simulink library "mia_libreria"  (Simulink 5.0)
undefined symbols (not defined in the file or in its folder): contributo_inerzia, coriolis, gravload, ikine_rrprrr, ikine_rrprrr1, interp_cubica, interp_grado5, interp_punti_intermedi, matrice2vettore, spazio_di_lavoro, stanf, verifica_assestamento, vettore2matrice, xyzrpr2tr
libraries: mia_libreria x11, roblocks x2, simulink x1

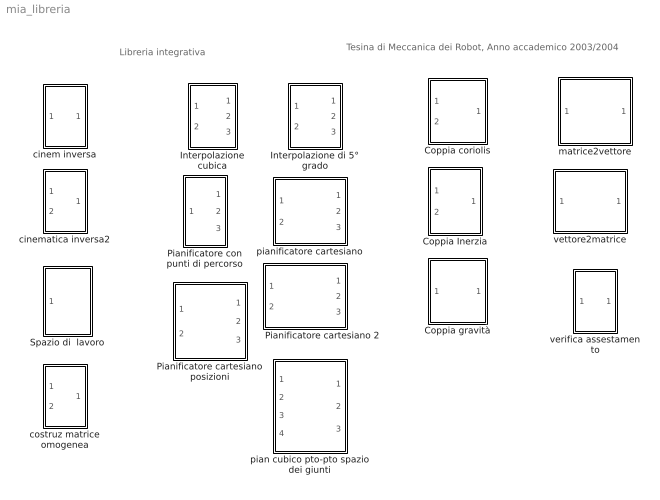
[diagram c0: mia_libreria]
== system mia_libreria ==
  note: Libreria integrativa
  note: Tesina di Meccanica dei Robot, Anno accademico 2003/2004
  Coppia Inerzia : Subsystem  mask{robot=0}
      mask prompts: robot "nome robot"
  Coppia coriolis : Subsystem  mask{robot=nome robot}
      mask prompts: robot "Variabile robot"
  Coppia gravità : Subsystem  mask{robot=0}
      mask prompts: robot "nome robot"
  Interpolazione cubica : Subsystem  mask{n=6, tf=1}
      mask prompts: n "dimensione uscita"; tf "tempo finale"
  Interpolazione di 5° grado : Subsystem  mask{n=0, tf=0}
      mask prompts: n "dimensione uscita"; tf "tempo finale"
  Pianificatore cartesiano 2 : Subsystem  mask{robot=0}
      mask prompts: robot "nome robot"
  Pianificatore cartesiano posizioni : Subsystem  mask{robot=stanf}
      mask prompts: robot "nome robot"
      mask help: funziona solo con manipolatori in cui il posizionamento dipende solo dalle variabili q1,q2,q3 e l'orientamento solo dalle variabili q4,q5,q6
  Pianificatore con punti di percorso : Subsystem  mask{robot=stanf, n_punti=2}
      mask prompts: robot "nome robot"; n_punti "numero punti traiettoria"
  Spazio di  lavoro : Subsystem  mask{robot=0}
      mask prompts: robot "nome robot"
  cinem inversa : Subsystem  mask{robot=stanf}
  cinematica inversa2 : Subsystem  mask{robot=stanf}
      mask prompts: robot "nome robot"
  costruz matrice omogenea : Subsystem
  matrice2vettore : Subsystem  mask{n_elementi=4}
      mask prompts: n_elementi "numero elementi della matrice"
  pian cubico pto-pto spazio dei giunti : Subsystem  mask{robot=0, tf=0}
      mask prompts: robot "nome robot"; tf "tempo finale"
  pianificatore cartesiano : Subsystem  mask{robot=0}
      mask prompts: robot "nome robot"
  verifica assestamento : Subsystem  mask{robot=stanf, vregime=1, scostpercentuale=0.1}
      mask prompts: robot "nome robot"; vregime "valore di regime desiderato"; scostpercentuale "scostamento dal valore di regime"
  vettore2matrice : Subsystem  mask{n_righe=2, n_colonne=2}
      mask prompts: n_righe "numero righe matrice uscita"; n_colonne "numero colonne matrice uscita"

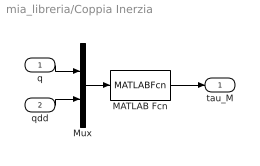
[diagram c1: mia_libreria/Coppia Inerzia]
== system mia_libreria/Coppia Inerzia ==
  q : Inport  PortDimensions=robot.n
  qdd : Inport  Port=2  PortDimensions=robot.n
  MATLAB Fcn : MATLABFcn  MATLABFcn=contributo_inerzia(robot,u(1:robot.n)',u(robot.n+1:2*robot.n)')  OutputDimensions=robot.n
  Mux : Mux  Inputs=2
  tau_M : Outport
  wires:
  Mux/1 -> MATLAB Fcn/1
  MATLAB Fcn/1 -> tau_M/1
  qdd/1 -> Mux/2
  q/1 -> Mux/1

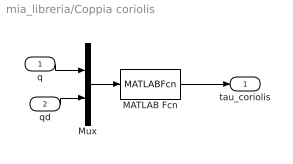
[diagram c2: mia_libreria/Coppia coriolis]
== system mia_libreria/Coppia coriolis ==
  q : Inport
  qd : Inport  Port=2
  MATLAB Fcn : MATLABFcn  MATLABFcn=coriolis(robot,u(1:robot.n)',u(robot.n+1:2*robot.n)')  OutputDimensions=robot.n
  Mux : Mux  Inputs=2
  tau_coriolis : Outport
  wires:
  Mux/1 -> MATLAB Fcn/1
  MATLAB Fcn/1 -> tau_coriolis/1
  qd/1 -> Mux/2
  q/1 -> Mux/1

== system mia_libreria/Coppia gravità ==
  q : Inport  PortDimensions=robot.n
  MATLAB Fcn : MATLABFcn  MATLABFcn=gravload(robot,u')  OutputDimensions=robot.n
  tau_grav : Outport
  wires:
  MATLAB Fcn/1 -> tau_grav/1
  q/1 -> MATLAB Fcn/1

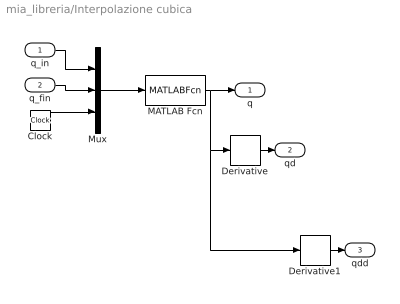
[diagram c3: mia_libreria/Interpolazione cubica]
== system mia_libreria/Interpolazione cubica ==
  q_in : Inport
  q_fin : Inport  Port=2
  Clock : Clock
  Derivative : Derivative
  Derivative1 : Derivative
  MATLAB Fcn : MATLABFcn  MATLABFcn=interp_cubica(u(1:n),u(n+1:2*n),tf,u(2*n+1))  OutputDimensions=n
  Mux : Mux  Inputs=3
  q : Outport
  qd : Outport  Port=2
  qdd : Outport  Port=3
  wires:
  MATLAB Fcn/1 -> q/1, Derivative/1, Derivative1/1
  q_in/1 -> Mux/1
  q_fin/1 -> Mux/2
  Clock/1 -> Mux/3
  Mux/1 -> MATLAB Fcn/1
  Derivative/1 -> qd/1
  Derivative1/1 -> qdd/1

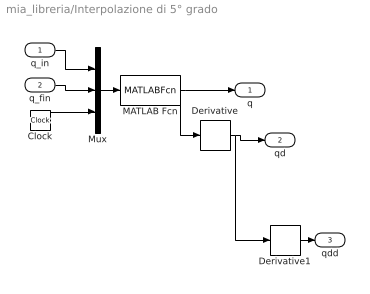
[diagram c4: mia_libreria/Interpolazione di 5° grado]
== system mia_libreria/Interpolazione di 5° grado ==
  q_in : Inport
  q_fin : Inport  Port=2
  Clock : Clock
  Derivative : Derivative
  Derivative1 : Derivative
  MATLAB Fcn : MATLABFcn  MATLABFcn=interp_grado5(u(1:n),u(n+1:2*n),tf,u(2*n+1))  OutputDimensions=n
  Mux : Mux  Inputs=3
  q : Outport
  qd : Outport  Port=2
  qdd : Outport  Port=3
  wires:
  Mux/1 -> MATLAB Fcn/1
  Clock/1 -> Mux/3
  q_fin/1 -> Mux/2
  q_in/1 -> Mux/1
  MATLAB Fcn/1 -> q/1, Derivative/1
  Derivative/1 -> qd/1, Derivative1/1
  Derivative1/1 -> qdd/1

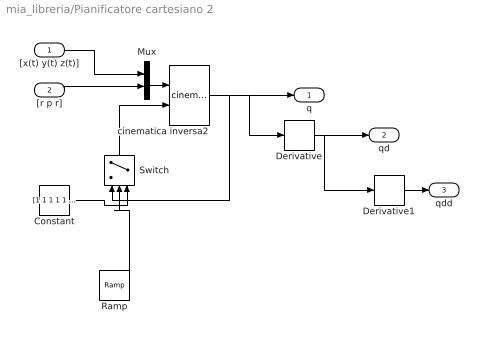
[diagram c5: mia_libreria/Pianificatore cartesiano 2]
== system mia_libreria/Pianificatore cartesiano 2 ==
  "[x(t) y(t) z(t)]" : Inport
  "[r p r]" : Inport  Port=2
  Constant : Constant  Value=[1 1 1 1 1 1]
  Derivative : Derivative
  Derivative1 : Derivative
  Mux : Mux  Inputs=2
  Ramp : simulink/Sources/Ramp  slope=1  start=0  X0=0
  Switch : Switch  Orientation=up  Threshold=1
  cinematica inversa2 : mia_libreria/cinematica inversa2  robot=stanf
  q : Outport
  qd : Outport  Port=2
  qdd : Outport  Port=3
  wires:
  Mux/1 -> cinematica inversa2/1
  "[r p r]"/1 -> Mux/2
  "[x(t) y(t) z(t)]"/1 -> Mux/1
  Derivative1/1 -> qdd/1
  Derivative/1 -> Derivative1/1, qd/1
  cinematica inversa2/1 -> Derivative/1, q/1, Switch/1
  Ramp/1 -> Switch/2
  Switch/1 -> cinematica inversa2/2
  Constant/1 -> Switch/3

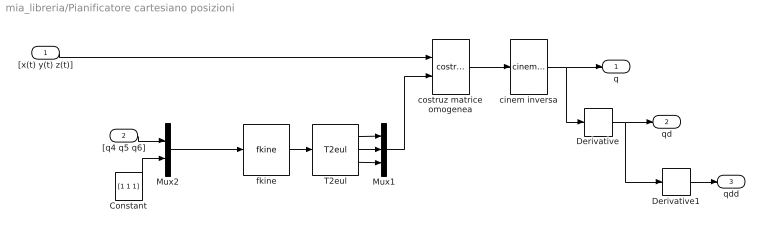
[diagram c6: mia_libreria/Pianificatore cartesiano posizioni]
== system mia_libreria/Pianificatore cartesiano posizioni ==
  "[x(t) y(t) z(t)]" : Inport
  "[q4 q5 q6]" : Inport  Port=2
  Constant : Constant  Value=[1 1 1]
  Derivative : Derivative
  Derivative1 : Derivative
  Mux1 : Mux  Inputs=3
  Mux2 : Mux  Inputs=2
  T2eul : roblocks/T2eul
  cinem inversa : mia_libreria/cinem inversa  robot=robot
  costruz matrice omogenea : mia_libreria/costruz matrice omogenea  SimViewingDevice=off  DataTypeOverride=UseLocalSettings  MinMaxOverflowLogging=UseLocalSettings
  fkine : roblocks/fkine  robot=robot
  q : Outport
  qd : Outport  Port=2
  qdd : Outport  Port=3
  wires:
  cinem inversa/1 -> q/1, Derivative/1
  Mux2/1 -> fkine/1
  Constant/1 -> Mux2/2
  "[q4 q5 q6]"/1 -> Mux2/1
  costruz matrice omogenea/1 -> cinem inversa/1
  Mux1/1 -> costruz matrice omogenea/2
  T2eul/3 -> Mux1/3
  T2eul/2 -> Mux1/2
  T2eul/1 -> Mux1/1
  fkine/1 -> T2eul/1
  "[x(t) y(t) z(t)]"/1 -> costruz matrice omogenea/1
  Derivative/1 -> qd/1, Derivative1/1
  Derivative1/1 -> qdd/1

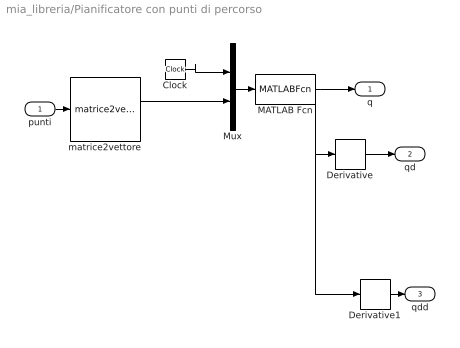
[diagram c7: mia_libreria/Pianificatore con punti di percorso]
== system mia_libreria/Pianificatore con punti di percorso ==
  punti : Inport
  Clock : Clock
  Derivative : Derivative
  Derivative1 : Derivative
  MATLAB Fcn : MATLABFcn  MATLABFcn=interp_punti_intermedi(vettore2matrice(u(2:n_punti*(2*robot.n+1)+1),n_punti,2*robot.n+1),u(1),robot.n)  OutputDimensions=robot.n  Output1D=off
  Mux : Mux  Inputs=2
  matrice2vettore : mia_libreria/matrice2vettore  n_elementi=n_punti*(2*robot.n+1)
  q : Outport
  qd : Outport  Port=2
  qdd : Outport  Port=3
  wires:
  Clock/1 -> Mux/1
  punti/1 -> matrice2vettore/1
  matrice2vettore/1 -> Mux/2
  Mux/1 -> MATLAB Fcn/1
  MATLAB Fcn/1 -> q/1, Derivative/1, Derivative1/1
  Derivative/1 -> qd/1
  Derivative1/1 -> qdd/1

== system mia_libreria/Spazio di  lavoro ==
  vincoli qi : Inport
  MATLAB Fcn : MATLABFcn  MATLABFcn=spazio_di_lavoro(u,robot)  Output1D=off
  Terminator : Terminator
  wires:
  vincoli qi/1 -> MATLAB Fcn/1
  MATLAB Fcn/1 -> Terminator/1

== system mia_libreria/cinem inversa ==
  T : Inport  PortDimensions=[4 4]
  MATLAB Fcn : MATLABFcn  MATLABFcn=ikine_rrprrr(robot,u)  OutputDimensions=robot.n
  q : Outport
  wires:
  T/1 -> MATLAB Fcn/1
  MATLAB Fcn/1 -> q/1

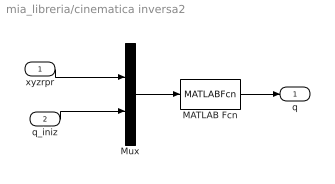
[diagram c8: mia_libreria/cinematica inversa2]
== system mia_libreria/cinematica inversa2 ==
  xyzrpr : Inport
  q_iniz : Inport  Port=2
  MATLAB Fcn : MATLABFcn  MATLABFcn=ikine_rrprrr1(robot,xyzrpr2tr(u(1),u(2),u(3),u(4),u(5),u(6)),u(7:6+robot.n))  OutputDimensions=robot.n
  Mux : Mux  Inputs=2
  q : Outport
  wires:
  xyzrpr/1 -> Mux/1
  Mux/1 -> MATLAB Fcn/1
  q_iniz/1 -> Mux/2
  MATLAB Fcn/1 -> q/1

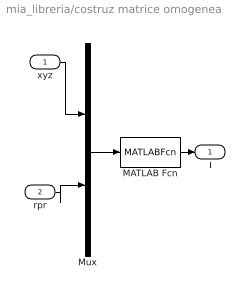
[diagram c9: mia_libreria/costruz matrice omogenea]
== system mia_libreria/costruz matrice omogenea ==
  xyz : Inport
  rpr : Inport  Port=2
  MATLAB Fcn : MATLABFcn  MATLABFcn=xyzrpr2tr(u(1),u(2),u(3),u(4),u(5),u(6))  OutputDimensions=[4 4]  Output1D=off
  Mux : Mux  Inputs=2
  T : Outport
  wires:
  rpr/1 -> Mux/2
  MATLAB Fcn/1 -> T/1
  Mux/1 -> MATLAB Fcn/1
  xyz/1 -> Mux/1

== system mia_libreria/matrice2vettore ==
  matrice : Inport
  MATLAB Fcn : MATLABFcn  MATLABFcn=matrice2vettore(u)  OutputDimensions=n_elementi  Output1D=off
  vettore : Outport
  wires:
  matrice/1 -> MATLAB Fcn/1
  MATLAB Fcn/1 -> vettore/1

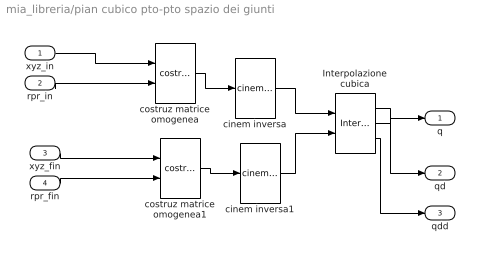
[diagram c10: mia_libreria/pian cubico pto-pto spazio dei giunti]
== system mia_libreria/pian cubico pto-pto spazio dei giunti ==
  xyz_in : Inport
  rpr_in : Inport  Port=2
  xyz_fin : Inport  Port=3
  rpr_fin : Inport  Port=4
  Interpolazione cubica : mia_libreria/Interpolazione cubica  robot=stanf  tf=tf
  cinem inversa : mia_libreria/cinem inversa  robot=stanf
  cinem inversa1 : mia_libreria/cinem inversa  robot=stanf
  costruz matrice omogenea : mia_libreria/costruz matrice omogenea  SimViewingDevice=off  DataTypeOverride=UseLocalSettings  MinMaxOverflowLogging=UseLocalSettings
  costruz matrice omogenea1 : mia_libreria/costruz matrice omogenea  SimViewingDevice=off  DataTypeOverride=UseLocalSettings  MinMaxOverflowLogging=UseLocalSettings
  q : Outport
  qd : Outport  Port=2
  qdd : Outport  Port=3
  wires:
  Interpolazione cubica/1 -> q/1
  cinem inversa/1 -> Interpolazione cubica/1
  cinem inversa1/1 -> Interpolazione cubica/2
  xyz_in/1 -> costruz matrice omogenea/1
  rpr_in/1 -> costruz matrice omogenea/2
  xyz_fin/1 -> costruz matrice omogenea1/1
  rpr_fin/1 -> costruz matrice omogenea1/2
  costruz matrice omogenea/1 -> cinem inversa/1
  costruz matrice omogenea1/1 -> cinem inversa1/1
  Interpolazione cubica/2 -> qd/1
  Interpolazione cubica/3 -> qdd/1

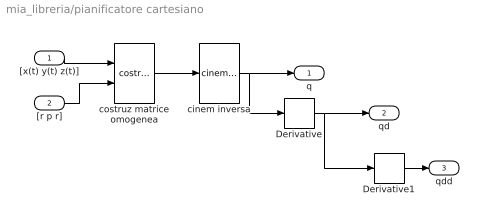
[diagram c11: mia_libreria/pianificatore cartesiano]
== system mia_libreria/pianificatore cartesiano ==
  "[x(t) y(t) z(t)]" : Inport
  "[r p r]" : Inport  Port=2
  Derivative : Derivative
  Derivative1 : Derivative
  cinem inversa : mia_libreria/cinem inversa  robot=robot
  costruz matrice omogenea : mia_libreria/costruz matrice omogenea  SimViewingDevice=off  DataTypeOverride=UseLocalSettings  MinMaxOverflowLogging=UseLocalSettings
  q : Outport
  qd : Outport  Port=2
  qdd : Outport  Port=3
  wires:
  Derivative1/1 -> qdd/1
  Derivative/1 -> Derivative1/1, qd/1
  "[r p r]"/1 -> costruz matrice omogenea/2
  cinem inversa/1 -> Derivative/1, q/1
  costruz matrice omogenea/1 -> cinem inversa/1
  "[x(t) y(t) z(t)]"/1 -> costruz matrice omogenea/1

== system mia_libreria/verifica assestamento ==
  in : Inport
  MATLAB Fcn : MATLABFcn  MATLABFcn=verifica_assestamento(u,vregime,scostpercentuale)  OutputDimensions=robot.n  Output1D=off
  test : Outport
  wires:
  MATLAB Fcn/1 -> test/1
  in/1 -> MATLAB Fcn/1

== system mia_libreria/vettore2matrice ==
  vettore : Inport
  MATLAB Fcn : MATLABFcn  MATLABFcn=vettore2matrice(u,n_righe,n_colonne)  OutputDimensions=[n_righe n_colonne]  Output1D=off
  matrice : Outport
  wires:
  vettore/1 -> MATLAB Fcn/1
  MATLAB Fcn/1 -> matrice/1
